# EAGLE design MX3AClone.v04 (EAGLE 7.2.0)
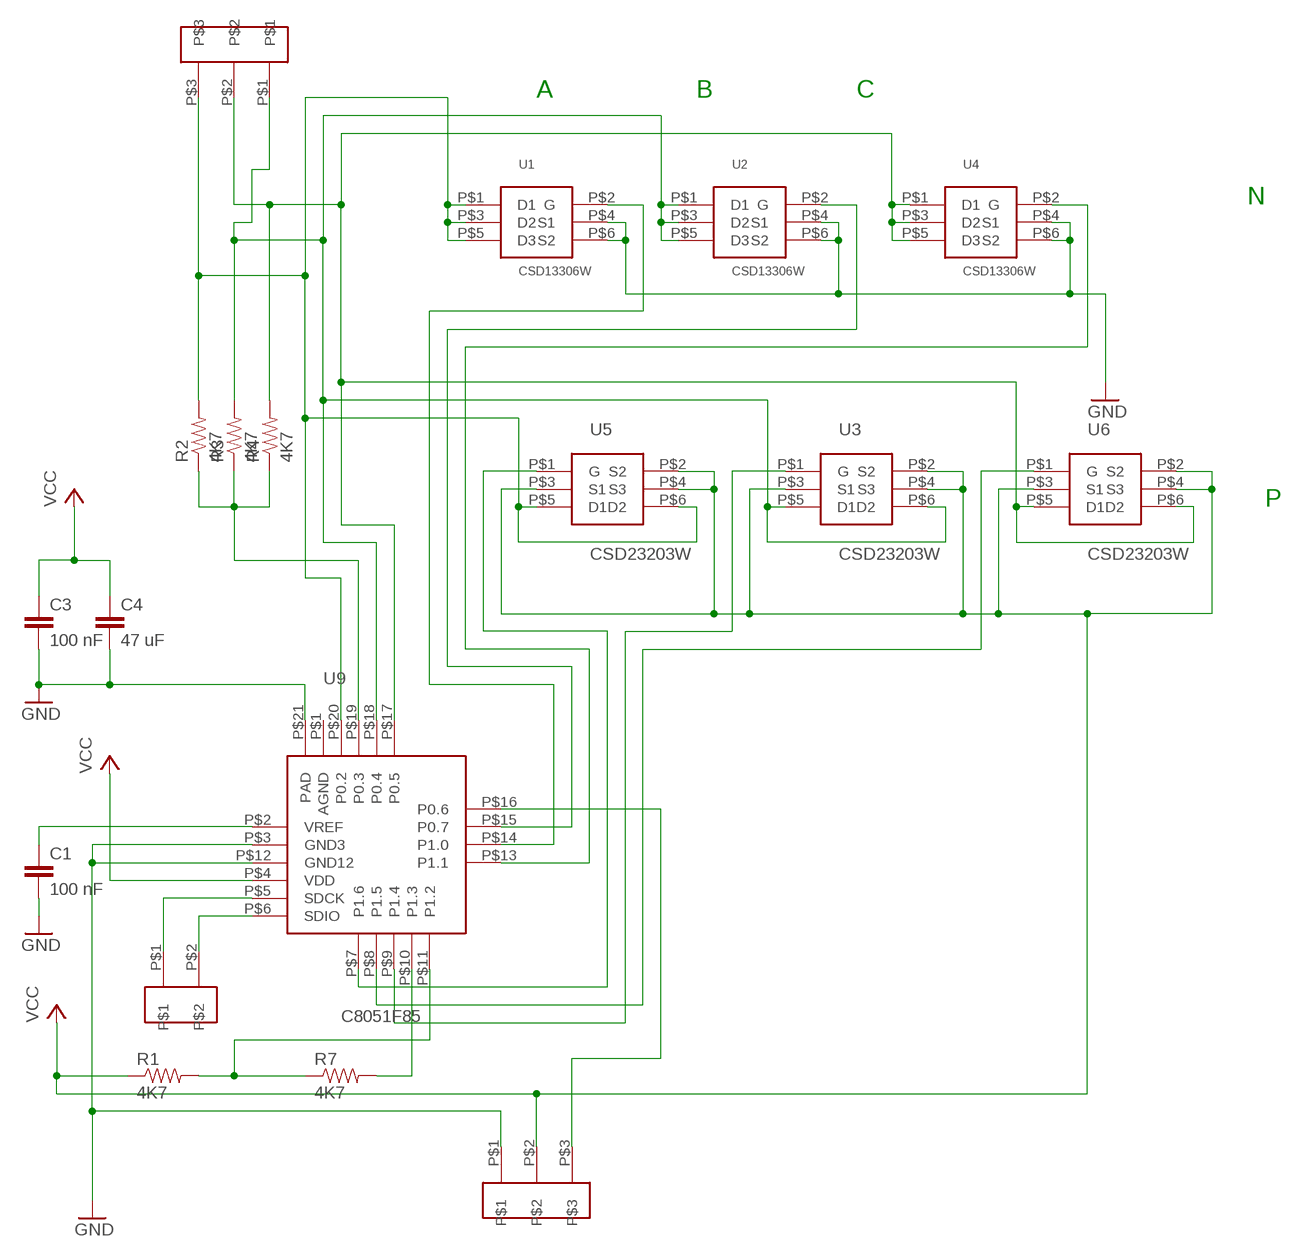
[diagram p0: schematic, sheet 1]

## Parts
C1  100 nF  0402CAP.KW  [0402-CAP]
C3  100 nF  0402CAP.KW  [0402-CAP]
C4  47 uF  0402CAP.KW  [0402-CAP]
R1  4K7  0402RES.KW  [0402-RES]
R2  4K7  0402RES.KW  [0402-RES]
R3  4K7  0402RES.KW  [0402-RES]
R4  4K7  0402RES.KW  [0402-RES]
R7  4K7  0402RES.KW  [0402-RES]
U1  CSD13306W  [CSD13306W]
U2  CSD13306W  [CSD13306W]
U3  CSD23203W  [CSD232203W]
U4  CSD13306W  [CSD13306W]
U5  CSD23203W  [CSD232203W]
U6  CSD23203W  [CSD232203W]
U9  C8051F85  [C8015F85]
U$1  HN02  [HN02]
U$2  HM03  [HM03]
U$4  HM03  [HM03]

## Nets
GND: C1.2 C3.2 C4.2 U1.P$4(S1) U1.P$6(S2) U2.P$4(S1) U2.P$6(S2) U4.P$4(S1) U4.P$6(S2) U9.P$3(GND3) U9.P$12(GND12) U9.P$21(PAD) U$4.P$1
N$1: U1.P$2(G) U9.P$14(P1.0)
N$2: U2.P$2(G) U9.P$15(P0.7)
N$3: U4.P$2(G) U9.P$13(P1.1)
N$4: U5.P$1(G) U9.P$7(P1.6)
N$5: U3.P$1(G) U9.P$9(P1.4)
N$6: U6.P$1(G) U9.P$8(P1.5)
N$7: R2.1 R3.1 R4.1 U9.P$19(P0.3)
N$9: R3.2 U2.P$1(D1) U2.P$3(D2) U2.P$5(D3) U3.P$5(D1) U3.P$6(D2) U9.P$18(P0.4) U$2.P$1
N$10: R4.2 U4.P$1(D1) U4.P$3(D2) U4.P$5(D3) U6.P$5(D1) U6.P$6(D2) U9.P$17(P0.5) U$2.P$2
N$11: C1.1 U9.P$2(VREF)
N$12: R7.2 U9.P$10(P1.3)
N$13: U9.P$6(SDIO) U$1.P$2
N$14: U9.P$5(SDCK) U$1.P$1
N$16: U9.P$16(P0.6) U$4.P$3
N$17: R1.2 R7.1 U9.P$11(P1.2)
N$18: R2.2 U1.P$1(D1) U1.P$3(D2) U1.P$5(D3) U5.P$5(D1) U5.P$6(D2) U9.P$20(P0.2) U$2.P$3
VCC: C3.1 C4.1 R1.1 U3.P$2(S2) U3.P$3(S1) U3.P$4(S3) U5.P$2(S2) U5.P$3(S1) U5.P$4(S3) U6.P$2(S2) U6.P$3(S1) U6.P$4(S3) U9.P$4(VDD) U$4.P$2

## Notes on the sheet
- A | B | C
- N
- P

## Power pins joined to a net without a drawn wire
AGND: U9.P$1(AGND)

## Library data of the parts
C1 C3 C4 = SparkFun-Capacitors:0402CAP.KW
R1-R4 R7 = SparkFun-Resistors:0402RES.KW
U1 U2 U4 = Kris:CSD13306W: DSBGA package for CSD13306W 12 V N-type NextFET
U3 U5 U6 = Kris:CSD23203W: DSBGA package for CSD23203W 8 V P-type NextFET
U9 = Kris:C8051F85: C8051F85 Silicon Labs 8-bit microcontroller
U$1 = Kris:HN02: 0.1 inch header
U$2 U$4 = Kris:HM03

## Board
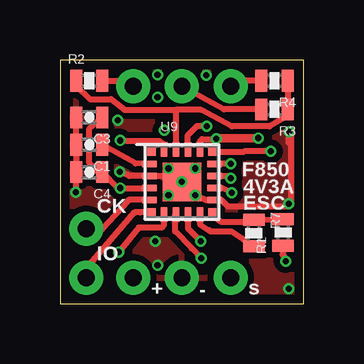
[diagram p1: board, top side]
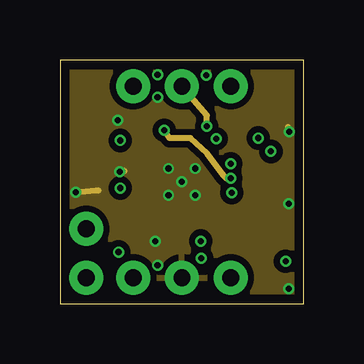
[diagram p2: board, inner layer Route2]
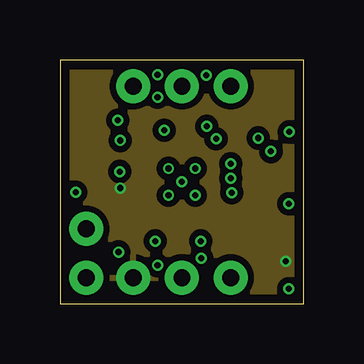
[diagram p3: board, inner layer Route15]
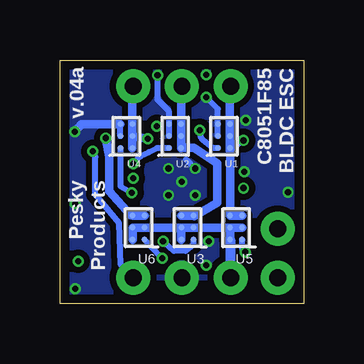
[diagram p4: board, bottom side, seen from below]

Size 10.16 x 10.16 mm. Coordinates in mm from the lower left corner, seen from the top.
Outline: 0,0 10.16,0 10.16,10.16 0,10.16 0,0
Copper layers (1*2*15*16): Top 0.035559375mm / dielectric 0.17018125mm / Route2 0.01778125mm / dielectric 47mil / Route15 0.01778125mm / dielectric 0.17018125mm / Bottom 0.035559375mm
Design rules "OSHPark-4layer *": minimum track width 5mil, minimum drill 10mil, track to track 5mil, track to pad 5mil, pad to pad 5mil, via to via 5mil, smd to smd 5mil, copper to edge 15mil, drill to drill 6mil, minimum pad ring 4mil, minimum via ring 4mil, stop-mask expansion 4mil, vias tented up to drill 20mil, thermal gap 10mil

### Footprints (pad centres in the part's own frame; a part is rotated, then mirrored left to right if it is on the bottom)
0402-CAP = smd 0.5 x 0.9: 1 -0.55,0; 2 0.55,0
0402-RES = smd 0.5 x 0.9: 1 -0.55,0; 2 0.55,0
CSD13306W = smd 0.26 x 0.26: P$1 -0.25,0.5; P$2 0.25,0.5; P$3 -0.25,0; P$4 0.25,0; P$5 -0.25,-0.5; P$6 0.25,-0.5
CSD232203W = smd 0.26 x 0.26: P$1 -0.25,0.5; P$2 0.25,0.5; P$3 -0.25,0; P$4 0.25,0; P$5 -0.25,-0.5; P$6 0.25,-0.5
C8015F85 = smd 0.34 x 0.34: P$1 -1.265,1.265; P$6 -1.265,-1.265; P$11 1.265,-1.265; P$16 1.265,1.265 | smd 0.61 x 0.28: P$2 -1.351,0.75; P$3 -1.351,0.25; P$4 -1.351,-0.25; P$5 -1.351,-0.75; P$12 1.351,-0.75; P$13 1.351,-0.25; P$14 1.351,0.25; P$15 1.351,0.75 | smd 0.28 x 0.61: P$7 -0.75,-1.351; P$8 -0.25,-1.351; P$9 0.25,-1.351; P$10 0.75,-1.351; P$17 0.75,1.351; P$18 0.25,1.351; P$19 -0.25,1.351; P$20 -0.75,1.351 | smd 1.6 x 1.6: P$21 0,0
HN02 = drill 0.7 pad 1.422: P$1 0,0; P$2 -2.032,0
HM03 = drill 0.7 pad 1.422: P$1 0,0; P$2 -2.032,0; P$3 2.032,0

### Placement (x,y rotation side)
C1  1.22,6.63 180 top
C3  1.22,7.77 180 top
C4  1.22,5.49 180 top
R1  9.3,2.97 90 top
R2  1.22,9.3 0 top
R3  8.94,8.1 180 top
R4  8.94,9.3 180 top
R7  8.08,2.95 270 top
U1  3.33,6.99 180 bottom
U2  5.36,6.99 180 bottom
U3  4.85,3.17 180 bottom
U4  7.39,6.99 180 bottom
U5  2.82,3.17 180 bottom
U6  6.88,3.17 180 bottom
U9  5.08,5.08 0 top
U$1  1.09,3.12 90 top
U$2  5.08,9.07 180 top
U$4  5.08,1.09 0 top

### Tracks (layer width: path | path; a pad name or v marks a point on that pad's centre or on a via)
GND  (via drill 0.25)
  Top 0.203: U9.P$12 6.72,4.33
  Top 0.254: v4.52,5.64 4.52,5.33 U9.P$3 2.9,5.33 v2.49,5.51 | 9.54,6.7 v9.55,7.16 | v0.66,4.65 0.67,5.43 C4.2 C1.2 C3.2 | v5.64,4.52 6.14,4.32 U9.P$12 | 6.72,4.33 6.99,4.06 9.53,4.06 9.63,4.17 9.63,7.14 9.58,7.19
  Route2 0.254: v9.55,7.16 9.5,7.37 | v0.66,4.65 1.5,4.72 1.6,4.72 | v2.49,5.51 2.69,5.54 2.67,5.54
  Bottom 0.203: 3.58,8.12 v4.06,8.61
  Bottom 0.254: 4.91,6.02 v4.52,5.64 | U1.P$4 U1.P$6 3.58,8.12 | U2.P$6 U2.P$4 5.61,8.02 6.1,8.51 v6.1,9.53 | U4.P$4 U4.P$6
  Bottom 0.356: U4.P$6 9.28,7.49 v9.55,7.16
  other vias: 5.64,5.64 4.52,4.52 5.08,5.08 4.06,9.55 9.53,4.17 2.41,7.65 4.06,1.6 3.96,2.62 9.53,0.64
  pour Top (isolate 0.254): 0,10.13 10.16,10.13 10.16,0 0,0
  pour Bottom (isolate 0.254): 0,10.16 10.16,10.16 10.16,0 0,0
  pour Route2 (isolate 0.254): 0,10.16 10.16,10.16 10.16,0 0,0
N$1  (via drill 0.25)
  Top 0.203: U9.P$14
  Top 0.254: U9.P$14 7.01,5.33 v7.11,5.23
  Route2 0.254: v7.11,5.23 6.93,5.23 6.78,5.38 6.12,6.27 5.44,6.91 4.57,6.91 v4.34,7.24
  Bottom 0.254: U1.P$2 3.77,6.49 4.19,6.81 4.27,6.91 v4.34,7.24
N$2  (via drill 0.25)
  Top 0.203: 6.44,5.84 U9.P$15
  Top 0.254: v7.11,5.84 6.44,5.84
  Bottom 0.254: U2.P$2 6.11,6.49 6.45,6.33 6.81,6.15 v7.11,5.84
N$3  (via drill 0.25)
  Top 0.254: U9.P$13 6.76,4.83 v7.16,4.62
  Bottom 0.203: 7.64,6.2
  Bottom 0.254: 7.64,6.2 7.64,4.9 v7.16,4.62 | U4.P$2 7.64,6.2
N$4  (via drill 0.25)
  Top 0.254: U9.P$7 4.33,3.29 4.24,3.17 3.28,3.17 v2.44,2.16
  Bottom 0.254: v2.44,2.16 2.56,2.29 U5.P$1
N$5  (via drill 0.25)
  Top 0.254: U9.P$9 5.33,3.15 v5.87,2.62
  Bottom 0.254: U3.P$1 4.6,2.46 4.93,2.21 5.41,2.21 v5.87,2.62
N$6  (via drill 0.25)
  Top 0.203: 4.8,3.7 U9.P$8
  Top 0.254: v5.89,1.91 5.49,2.31 4.8,3.02 4.8,3.7
  Bottom 0.254: U6.P$1 6.35,2.39 v5.89,1.91
N$7
  Top 0.254: R4.1 R3.1 9.49,7.84 8.74,7.39 7.16,7.39 5.89,8.08 4.83,8.08 | R2.1 0.67,9.06 1.25,8.53 2.13,8.53 2.69,8.08 4.83,8.08 | 4.83,8.08 U9.P$19
N$9  (via drill 0.25)
  Top 0.254: R3.2 6.83,8.1 U$2.P$1 | U9.P$18 5.33,7.03 5.71,7.42 6.1,7.42 v6.12,7.39
  Route2 0.254: v6.12,7.39 6.12,7.85 U$2.P$1
  Bottom 0.203: 5.11,9.04 U$2.P$1
  Bottom 0.254: U3.P$5 U3.P$6 | 4.67,3.67 4.65,3.66 4.57,3.66 | 5.09,6.5 U2.P$1
  Bottom 0.356: U2.P$1 U2.P$3 U2.P$5 5.11,9.04 | U3.P$6 4.67,3.67 | 4.57,3.66 3.61,4.22 3.61,5.87 4.6,6.5 5.09,6.5
N$10  (via drill 0.25)
  Top 0.254: R4.2 7.44,9.3 U$2.P$2 | U9.P$17 5.83,6.77 5.92,6.86 6.48,6.86 v6.5,6.88
  Top 0.356: v8.26,6.91 6.6,6.91 v6.5,6.88
  Bottom 0.203: 7.14,9.04 U$2.P$2
  Bottom 0.254: U6.P$6 7.16,3.69 7.22,3.69
  Bottom 0.356: U4.P$1 U4.P$3 | U4.P$3 U4.P$5 7.14,9.04 | U6.P$5 U6.P$6 | U4.P$3 v6.5,6.88 | 7.22,3.69 8.1,4.7 8.1,6.15 v8.26,6.91
N$11
  Top 0.254: U9.P$2 3.15,5.86 C1.1
N$12
  Top 0.254: U9.P$10 5.83,3.32 6.2,3.07 6.27,3.02 7.15,3.02 R7.2
N$13
  Top 0.254: U9.P$6 3.33,3.81 3.15,3.81 3.1,3.81 1.09,1.47 U$1.P$2
N$14
  Top 0.254: U9.P$5 2.86,4.33 2.86,4.3 1.75,3.1 1.12,3.1 U$1.P$1
N$16  (via drill 0.25)
  Top 0.254: U9.P$16 7.67,6.34 7.68,6.35 v8.79,6.35
  Bottom 0.254: v8.79,6.35 8.69,6.12 8.69,4.57 7.7,3.35 7.62,1.63 7.42,1.4 U$4.P$3
N$17
  Top 0.203: U9.P$11 6.34,3.71 | 8.04,3.43 R7.1
  Top 0.254: 6.34,3.71 6.71,3.43 8.04,3.43 | R7.1 R1.2
N$18  (via drill 0.25)
  Top 0.254: R2.2 2.82,9.3 U$2.P$3 | U9.P$20 4.33,6.67 4.14,6.78 2.77,6.78 v2.52,6.81
  Bottom 0.203: 3.08,9.04 U$2.P$3
  Bottom 0.254: v2.52,6.81 2.6,6.81
  Bottom 0.356: U1.P$1 U1.P$3 U1.P$5 3.08,9.04 | U5.P$5 U5.P$6 3.07,4.04 3.07,4.22 3.07,6.16 U1.P$1 | 2.6,6.81 2.82,6.66 U1.P$1
VCC  (via drill 0.25)
  Top 0.203: 3.66,4.83 U9.P$4
  Top 0.254: C3.1 1.22,7.3 1.22,5.87 1.6,5.49 C4.1 2.4,4.83 v2.52,4.83 3.66,4.83 | R1.1 9.27,2.06 v9.4,1.78
  Route15 0.203: v9.4,1.78 9.4,1.7
  Bottom 0.356: U5.P$3 U5.P$4 | U5.P$4 U3.P$3 U3.P$4 | U3.P$4 U3.P$2 | U3.P$4 U6.P$3 U6.P$4 U6.P$2 | U5.P$4 U5.P$2
  Bottom 0.406: U5.P$2 3.07,1.11 U$4.P$2
  pour Route15 (isolate 0.254): 0,10.16 10.16,10.16 10.16,0 0,0

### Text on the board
tPlace: F850 | 4V3A | CK | ESC | IO | + | - | s
bPlace: C8051F85 / BLDC ESC | v.04a | Pesky / Products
